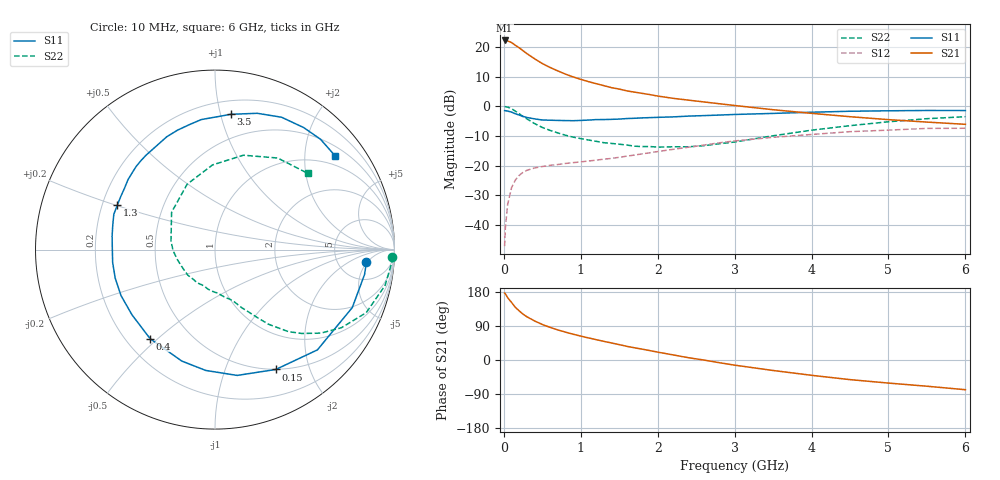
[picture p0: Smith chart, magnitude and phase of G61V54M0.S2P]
! SIEMENS Small Signal Semiconductors
! BFG193
! Si NPN RF Bipolar Junction Transistor in SOT223
! VCE = 1.5 V  IC = 4 mA
! Common Emitter S-Parameters:  August  1996
# GHz  S  MA  R  50
!  f  S11  S21  S12  S22
! GHz  MAG  ANG  MAG  ANG  MAG  ANG  MAG  ANG
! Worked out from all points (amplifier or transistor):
!   36 points, 10 MHz to 6 GHz, reference 50 ohm
!   highest |S21| = 22.2 dB at 10 MHz (marker M1)
!   |S21| within 3 dB of that: start of sweep to 226.5 MHz
!   unconditionally stable (mu >= 1): 1.186 GHz to 2.797 GHz
!   at 250 MHz: K = 0.30, MSG = 20.5 dB, |S12| = -22.2 dB
!   at 1.4 GHz: K = 1.10, MAG = 10.0 dB, |S12| = -17.6 dB
!   at 6 GHz: K = 0.95, MSG = 0.7 dB, |S12| = -7.4 dB
!   S11 on the Smith chart (normalised r, x): 10 MHz: 10, -5; 150 MHz: 0.50, -1.51; 400 MHz: 0.30, -0.47; 1.3 GHz: 0.26, +0.20; 3.5 GHz: 0.30, +1.08; 6 GHz: 0.73, +2.73
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0.01  0.8469 -4.7  12.87 176.8  0.0044 90.9  0.9897 -2.4
0.02  0.8446 -9.5  12.84 174.6  0.009 86.6  0.9853 -4.8
0.05  0.8303 -22.9  12.63 164.3  0.0224 78.6  0.9684 -11.9
0.1  0.7986 -44.4  11.86 152.0  0.0424 68.2  0.9131 -22.6
0.15  0.7488 -63.1  10.66 138.9  0.0574 58.2  0.8282 -31.7
0.2  0.7118 -80.0  9.669 129.6  0.0687 51.8  0.7509 -38.3
0.25  0.6752 -94.4  8.638 120.9  0.0773 46.0  0.6714 -44.1
0.3  0.648 -106.6  7.719 114.0  0.0835 42.1  0.613 -48.2
0.4  0.6139 -126.1  6.321 103.1  0.0915 36.4  0.5113 -54.4
0.5  0.5882 -141.8  5.248 93.7  0.0967 32.9  0.4401 -58.5
0.6  0.583 -154.0  4.517 86.2  0.1014 31.2  0.3931 -61.8
0.7  0.5783 -164.1  3.956 79.5  0.1045 30.1  0.357 -65.2
0.9  0.5721 179.4  3.132 68.1  0.1124 29.3  0.3024 -70.6
1.1  0.5861 166.3  2.604 58.3  0.1197 29.7  0.2706 -78.3
1.3  0.598 155.4  2.227 49.2  0.1288 30.1  0.2437 -85.8
1.6  0.622 141.2  1.818 36.0  0.1448 29.8  0.2224 -100.7
2.2  0.6632 119.5  1.363 13.5  0.1884 26.1  0.2079 -137.0
2.8  0.7118 101.2  1.105 -7.1  0.2425 18.0  0.2338 -178.7
3.5  0.7589 83.3  0.876 -27.7  0.3005 3.1  0.319 139.3
4.5  0.8255 63.3  0.668 -51.8  0.3739 -17.2  0.4719 91.7
5.5  0.8506 46.3  0.542 -69.2  0.4245 -42.1  0.6184 55.6
6  0.849 38.0  0.497 -78.4  0.4269 -56.1  0.6685 39.5
